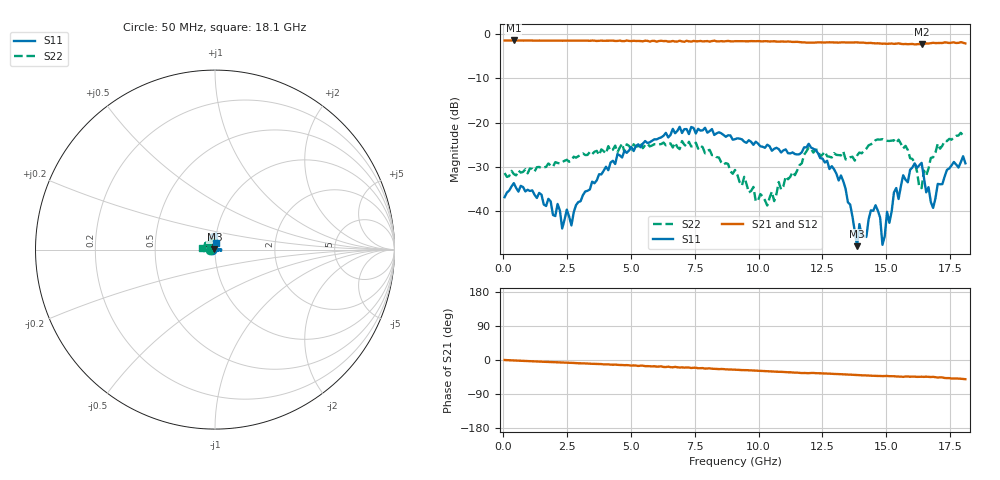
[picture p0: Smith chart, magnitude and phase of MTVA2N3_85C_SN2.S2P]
! Network Analyzer HP8720D.06.14 Serial No. US36140669
! 11 May 2005  12:56:36
! Frequency  S11  S21  S12  S22
# HZ  S  DB R 50
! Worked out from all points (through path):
!   201 points, 50 MHz to 18.1 GHz, reference 50 ohm
!   highest |S21| = -1.51 dB at 411 MHz (marker M1); lowest = -2.4 dB at 16.39 GHz (marker M2)
!   group delay of S21, straight-line fit = 7.69 ps
!   lowest |S11| = -47.8 dB at 13.86 GHz (marker M3), VSWR 1.01, Z = 49.7 + j0.201 ohm
!   |S11| at or under -10 dB: start of sweep to end of sweep
!   |S22| runs from -38.7 to -22.3 dB; largest |S21 - S12| = 0.027
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5e7  -36.80 -170.1  -1.53 -0.1  -1.53 -0.6  -31.37 -175.4
4.11e8  -33.65 -170.5  -1.51 -1.3  -1.51 -1.6  -31.61 -179.2
2.12575e9  -38.34 164.1  -1.54 -6.2  -1.55 -6.5  -29.11 157.7
2.30625e9  -43.87 165.8  -1.56 -6.6  -1.55 -7.0  -28.92 158.2
3.1185e9  -36.35 93.6  -1.56 -8.8  -1.57 -9.5  -26.96 152.4
6.09675e9  -23.53 86.3  -1.64 -17.3  -1.57 -17.6  -24.95 105.0
9.075e9  -23.75 112.5  -1.67 -25.6  -1.64 -26.1  -30.68 95.0
1.03385e10  -24.99 127.4  -1.69 -29.6  -1.68 -30.2  -38.70 138.5
1.21435e10  -25.91 132.4  -2.00 -34.1  -1.97 -34.8  -26.77 138.4
1.32265e10  -31.92 128.0  -1.96 -37.5  -1.96 -37.9  -27.39 135.2
1.385825e10  -47.85 150.0  -1.94 -39.6  -1.93 -40.3  -27.43 153.7
1.39485e10  -42.88 174.9  -2.01 -39.9  -1.96 -40.5  -26.76 158.3
1.421925e10  -45.77 -114.4  -2.10 -40.8  -2.07 -41.3  -25.90 163.7
1.458025e10  -38.63 -105.5  -2.16 -42.1  -2.06 -42.7  -23.97 155.7
1.4851e10  -47.55 -121.4  -2.24 -42.5  -2.18 -42.8  -23.74 146.8
1.50315e10  -40.12 -41.7  -2.26 -42.1  -2.22 -43.3  -24.12 143.2
1.512175e10  -42.58 -33.6  -2.24 -42.7  -2.16 -42.8  -24.15 140.6
1.53925e10  -34.75 -4.9  -2.23 -43.6  -2.16 -43.4  -24.59 136.1
1.638525e10  -29.09 -10.5  -2.42 -44.1  -2.28 -44.5  -34.77 149.7
1.68365e10  -39.23 57.5  -2.04 -44.5  -2.00 -45.9  -27.83 -171.1
1.7378e10  -30.66 81.0  -1.99 -47.8  -1.85 -48.8  -24.18 178.8
1.81e10  -29.18 83.8  -2.17 -50.6  -2.10 -52.1  -22.69 174.5
